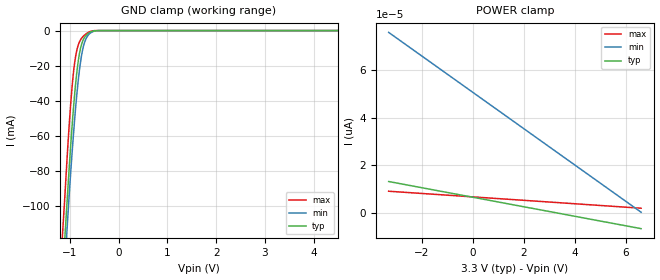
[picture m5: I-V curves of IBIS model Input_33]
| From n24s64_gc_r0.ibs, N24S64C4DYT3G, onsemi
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|//////////////////////////////////////////////////////////////////////////////
|//////////////////////////////////////////////////////////////////////////////
[Model]  Input_33
Model_type Input
Vinh = 2.31
Vinl = 0.99
|  variable   typ   min   max
C_comp   6pF   6pF   6pF
|//////////////////////////////////////////////////////////////////////////////
[Temperature Range]   25   85   -40
|//////////////////////////////////////////////////////////////////////////////
[Voltage Range]   3.30V   3.00V   3.60V
|//////////////////////////////////////////////////////////////////////////////
[POWER Clamp Reference] 3.30V   3.00V   3.60V
|//////////////////////////////////////////////////////////////////////////////
[GND Clamp Reference]   0V   0V   0V
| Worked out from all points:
|   GND clamp passes 1 mA (typ) near -0.59 V on its own axis
|//////////////////////////////////////////////////////////////////////////////
[GND Clamp]
|   Voltage   I(typ)   I(min)   I(max)
-3.3V     -1.107A    -1.122A    -1.083A
-1.18V    -152.4mA   -167.9mA   -128.8mA
-1.14V    -134.4mA   -149.9mA   -110.8mA
-1.1V     -116.4mA   -131.9mA   -92.78mA
-1.06V    -98.35mA   -113.9mA   -73.71mA
-1V       -72.14mA   -87.52mA   -48.02mA
-940mV    -48.84mA   -63.94mA   -27.48mA
-840mV    -19.69mA   -31.39mA   -9.219mA
-780mV    -9.859mA   -17.55mA   -5.183mA
-720mV    -4.897mA   -8.694mA   -3.11mA
-580mV    -874uA     -1.393mA   -508uA
6.6V      13.13pA    78.12pA    8.837pA
|//////////////////////////////////////////////////////////////////////////////
[POWER Clamp]
|   Voltage   I(typ)   I(min)   I(max)
-3.3V     13.13pA    75.83pA    9.054pA
0V        6.529pA    50.63pA    6.673pA
3.3V      -77.34fA   25.43pA    4.292pA
6.6V      -6.683pA   224.3fA    1.91pA
